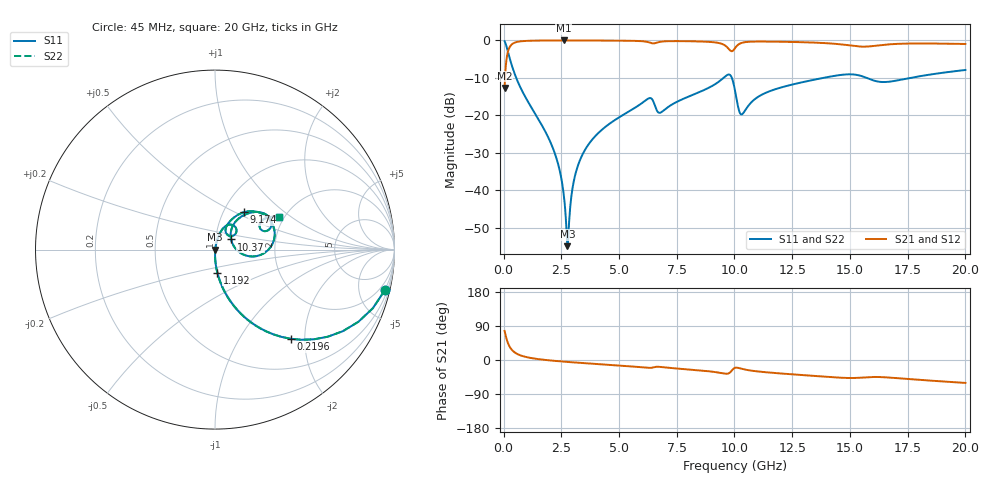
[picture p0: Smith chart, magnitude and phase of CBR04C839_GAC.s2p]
! S-parameter model data by Modelithics Inc.  support@modelithics.com 813-866-6335  Tampa FL USA
! S-Parameter data specifications:
! Substrate: 20-mil Rogers 4350B, substrate thickness, H=0.508mm, Dielectric constant, Er=3.75
! PCB Mounting Pad Footprint: Pad width, PadW=0.52mm , Pad length, PadL=0.52mm , Pad gap, PadG (edge-to-edge)=0.28mm , Reference planes=1.32mm apart
#  GHz  S  MA  R 50
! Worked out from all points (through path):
!   801 points, 45 MHz to 20 GHz, reference 50 ohm
!   highest |S21| = -0.02 dB at 2.614 GHz (marker M1); lowest = -12.7 dB at 45 MHz (marker M2)
!   group delay of S21, straight-line fit = 9.67 ps
!   lowest |S11| = -55.0 dB at 2.764 GHz (marker M3), VSWR 1.00, Z = 50.2 - j0.0524 ohm
!   |S11| at or under -10 dB: 547.2 MHz to 9.525 GHz (8.978 GHz wide, 178 % of centre); 9.885 GHz to 13.86 GHz (3.972 GHz wide, 33.5 % of centre); 15.72 GHz to 17.63 GHz (1.916 GHz wide, 11.5 % of centre)
!   |S22| runs from -55.0 to -0.2 dB; largest |S21 - S12| = 0
!   S11 on the Smith chart (normalised r, x): 45 MHz: 0.99, -8.38; 219.6 MHz: 0.99, -1.71; 1.192 GHz: 0.99, -0.26; 9.174 GHz: 1.24, +0.55; 10.37 GHz: 1.19, +0.14; 20 GHz: 1.89, +0.82
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0.045  0.973 -13.4  0.2308 76.6  0.2308 76.6  0.973 -13.4
0.219606  0.6514 -49.7  0.7583 40.2  0.7583 40.2  0.6514 -49.7
0.518931  0.3328 -71.4  0.9422 18.5  0.9422 18.5  0.3328 -71.4
1.192413  0.1289 -84.3  0.9905 5.2  0.9905 5.2  0.1289 -84.3
2.190163  0.0329 -89.4  0.9978 -2.1  0.9978 -2.1  0.0329 -89.4
2.4396  0.01782 -88.2  0.9981 -3.5  0.9981 -3.5  0.01782 -88.2
2.614206  0.008301 -82.5  0.9982 -4.3  0.9982 -4.3  0.008301 -82.5
2.763869  0.001787 -17.0  0.9982 -5.1  0.9982 -5.1  0.001787 -17.0
3.063194  0.0142 76.1  0.9979 -6.4  0.9979 -6.4  0.0142 76.1
3.387462  0.02861 78.2  0.9975 -7.9  0.9975 -7.9  0.02861 78.2
4.260494  0.06418 76.4  0.9954 -11.5  0.9954 -11.5  0.06418 76.4
6.23105  0.1647 57.8  0.954 -20.7  0.954 -20.7  0.1647 57.8
6.704981  0.1089 45.7  0.9465 -17.9  0.9465 -17.9  0.1089 45.7
9.174413  0.2617 52.5  0.9397 -31.9  0.9397 -31.9  0.2617 52.5
9.773062  0.3497 20.1  0.7556 -34.5  0.7556 -34.5  0.3497 20.1
10.0225  0.2142 -10.3  0.7881 -20.5  0.7881 -20.5  0.2142 -10.3
10.22205  0.1097 6.8  0.9019 -21.7  0.9019 -21.7  0.1097 6.8
10.37171  0.1062 32.4  0.9371 -24.1  0.9371 -24.1  0.1062 32.4
11.26969  0.1942 53.7  0.9654 -31.8  0.9654 -31.8  0.1942 53.7
13.36496  0.2948 44.8  0.9368 -41.6  0.9368 -41.6  0.2948 44.8
16.68248  0.2804 27.8  0.8855 -46.3  0.8855 -46.3  0.2804 27.8
20  0.4026 26.8  0.896 -60.5  0.896 -60.5  0.4026 26.8
